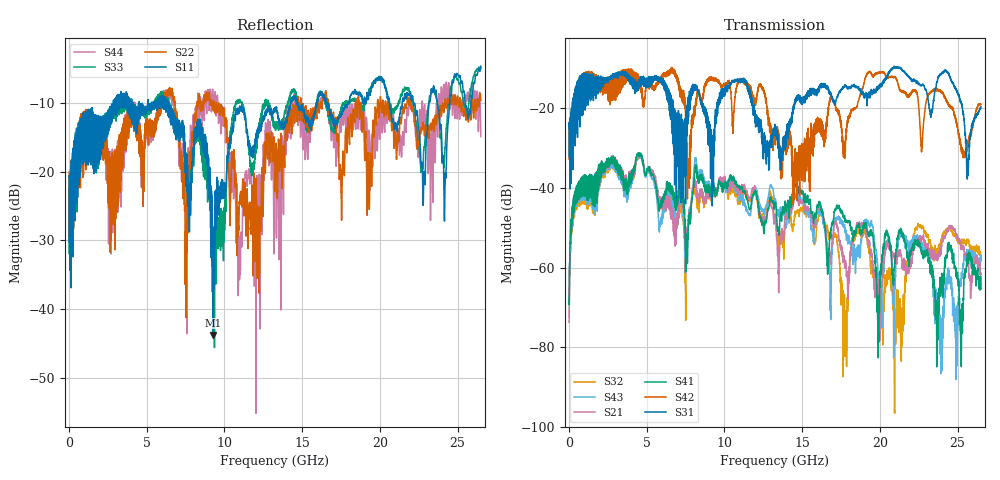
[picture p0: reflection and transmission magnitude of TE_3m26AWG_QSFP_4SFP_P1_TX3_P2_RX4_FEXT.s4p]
!Agilent Technologies,N5222A,MY51421691,A.10.00.00
!Agilent N5222A: A.10.00.00
!Date: Friday, January 30, 2015 12:38:17
!Correction: S11(Full 4 Port(1,2,3,4))
!S12(Full 4 Port(1,2,3,4))
!S13(Full 4 Port(1,2,3,4))
!S14(Full 4 Port(1,2,3,4))
!S21(Full 4 Port(1,2,3,4))
!S22(Full 4 Port(1,2,3,4))
!S23(Full 4 Port(1,2,3,4))
!S24(Full 4 Port(1,2,3,4))
!S31(Full 4 Port(1,2,3,4))
!S32(Full 4 Port(1,2,3,4))
!S33(Full 4 Port(1,2,3,4))
!S34(Full 4 Port(1,2,3,4))
!S41(Full 4 Port(1,2,3,4))
!S42(Full 4 Port(1,2,3,4))
!S43(Full 4 Port(1,2,3,4))
!S44(Full 4 Port(1,2,3,4))
!S4P File: Measurements: <S11,S12,S13,S14>,
!<S21,S22,S23,S24>,
!<S31,S32,S33,S34>,
!<S41,S42,S43,S44>:
# Hz S  dB  R 50.0
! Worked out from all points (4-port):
!   2650 points, 10 MHz to 26.5 GHz, reference 50 ohm
!   strongest paths, dB at 10 MHz, 6.63 GHz, 13.26 GHz, 19.88 GHz, 26.5 GHz:
!     S31: -25.0, -17.7, -24.7, -15.3, -19.6
!     S42: -25.0, -10.9, -25.2, -11.1, -19.0
!     S41: -68.4, -40.3, -43.6, -77.9, -65.3
!     S21: -73.7, -45.6, -46.5, -69.1, -61.6
!     S43: -72.4, -42.7, -42.7, -61.9, -58.0
!     S32: -68.1, -45.1, -47.0, -64.4, -57.7
!   lowest |S11| = -43.8 dB at 9.27 GHz (marker M1), VSWR 1.01, Z = 50 + j0.647 ohm
!   |S11| at or under -10 dB: start of sweep to 2.858 GHz; 6.4 GHz to 14.25 GHz (7.849 GHz wide, 76 % of centre); 16.59 GHz to 17.95 GHz (1.357 GHz wide, 7.86 % of centre)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
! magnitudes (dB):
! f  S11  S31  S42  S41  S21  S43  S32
! 10 MHz  -20.8  -25.0  -25.0  -68.4  -73.7  -72.4  -68.1
! 2.75 GHz  -10.2  -12.0  -12.5  -33.2  -33.0  -34.2  -34.2
! 9.27 GHz  -43.8  -27.7  -12.6  -39.4  -40.3  -38.8  -41.0
! 11 GHz  -11.2  -12.9  -12.8  -40.0  -41.1  -43.0  -44.1
! 16.24 GHz  -8.7  -13.7  -25.3  -45.5  -45.3  -46.6  -46.0
! 17.76 GHz  -10.4  -14.3  -28.2  -47.8  -59.0  -49.9  -73.0
! 26.5 GHz  -4.7  -19.6  -19.0  -65.3  -61.6  -58.0  -57.7
